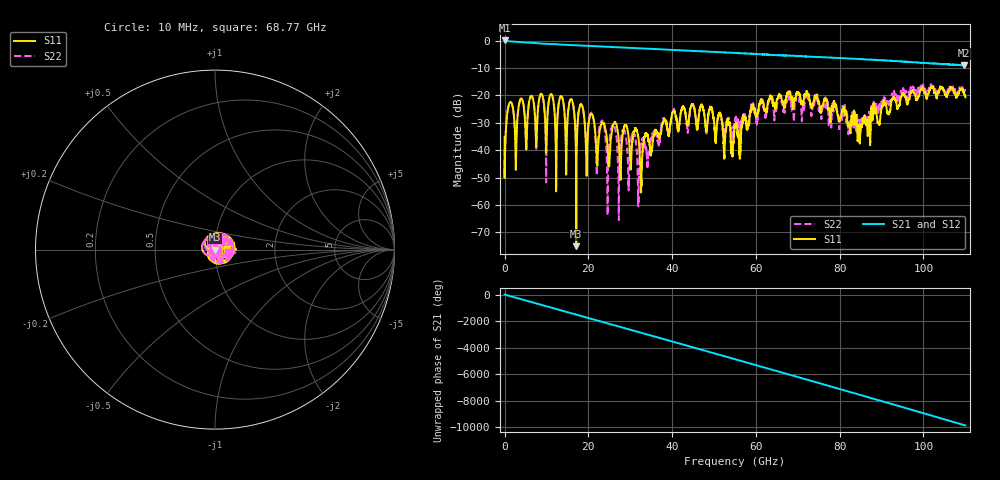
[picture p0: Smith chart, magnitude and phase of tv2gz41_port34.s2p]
!Keysight Technologies,N5247A,US51370218,A.10.49.08
!Posted to IEEE NEA 05/29  by John Calvin
!Date: Wednesday, February 21, 2018 15:43:19
!Correction: S11(Full 2 Port(1,2))
!S21(Full 2 Port(1,2))
!S12(Full 2 Port(1,2))
!S22(Full 2 Port(1,2))
!S2P File: Measurements: S11, S21, S12, S22:
# Hz S  dB  R 50
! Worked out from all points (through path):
!   11000 points, 10 MHz to 110 GHz, reference 50 ohm
!   highest |S21| = 0.08 dB at 10 MHz (marker M1); lowest = -9.0 dB at 109.7 GHz (marker M2)
!   group delay of S21, straight-line fit = 248 ps
!   lowest |S11| = -75.1 dB at 17.11 GHz (marker M3), VSWR 1.00, Z = 50 + j0.0131 ohm
!   |S11| at or under -10 dB: start of sweep to end of sweep
!   |S22| runs from -65.5 to -15.7 dB; largest |S21 - S12| = 0.0087
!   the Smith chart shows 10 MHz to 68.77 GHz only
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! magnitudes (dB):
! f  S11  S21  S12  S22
! 10 MHz  -35.1  0.1  0.1  -39.5
! 1.28 GHz  -22.5  -0.3  -0.3  -22.6
! 2.68 GHz  -47.2  -0.4  -0.4  -39.8
! 8.74 GHz  -19.3  -1.1  -1.1  -19.5
! 9.91 GHz  -40.5  -1.1  -1.1  -50.1
! 11.03 GHz  -19.5  -1.3  -1.3  -19.7
! 12.31 GHz  -55.1  -1.3  -1.3  -46.6
! 15.97 GHz  -21.4  -1.6  -1.6  -21.4
! 17.11 GHz  -75.1  -1.7  -1.7  -38.2
! 18.35 GHz  -23.3  -1.8  -1.8  -23.3
! 19.53 GHz  -45.6  -1.9  -1.9  -40.0
! 23.33 GHz  -30.0  -2.1  -2.2  -29.3
! 24.56 GHz  -38.3  -2.2  -2.2  -57.9
! 25.86 GHz  -30.9  -2.3  -2.3  -30.5
! 31.95 GHz  -35.5  -2.8  -2.8  -59.0
! 36.68 GHz  -34.9  -3.1  -3.1  -37.9
! 44.79 GHz  -23.2  -3.7  -3.7  -23.5
! 55.01 GHz  -31.2  -4.5  -4.5  -29.9
! 73.34 GHz  -24.4  -5.9  -5.9  -26.7
! 91.67 GHz  -27.0  -7.3  -7.3  -23.5
! 109.7 GHz  -19.4  -9.0  -9.0  -19.1
! 110 GHz  -20.7  -9.0  -9.0  -18.9
